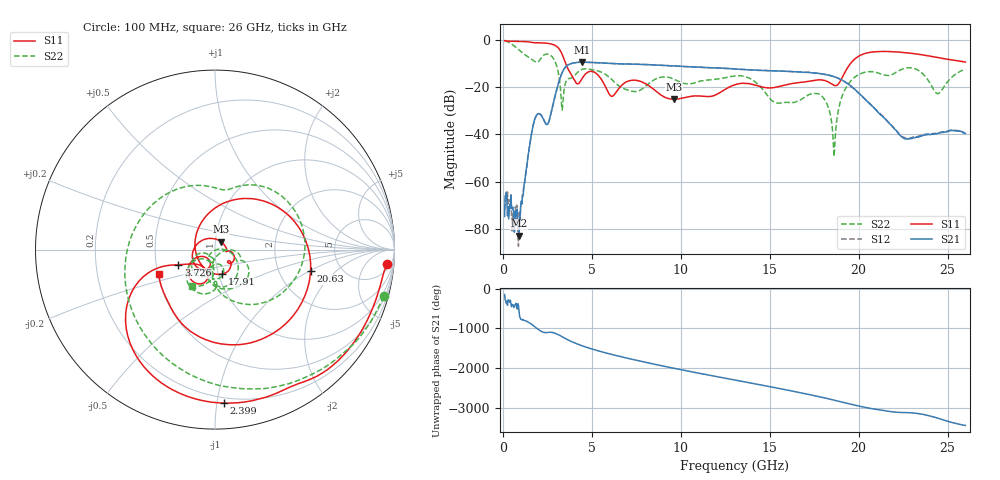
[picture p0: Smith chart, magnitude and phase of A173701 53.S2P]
!  2-Port S-parameters saved by WinCal
! VAR MeasName=S-Parameters (CALIBRATED_DATA) read from VNA (N5245A)
! VAR MeasDate=2017-6-7 10:31:55
! VAR NAME=A173701 53
! VAR FILENAME=A173701 53.S2P
! VAR DATE=2017-6-7 10:31:55
! VAR PHYS_PORTS=1,2
# Hz S DB R 50
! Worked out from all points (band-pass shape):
!   801 points, 100 MHz to 26 GHz, reference 50 ohm
!   highest |S21| = -9.40 dB at 4.438 GHz (marker M1); lowest = -83.0 dB at 909.4 MHz (marker M2)
!   |S21| within 3 dB of the highest: 3.435 GHz to 13.26 GHz (9.823 GHz wide, 118 % of centre)
!   lowest |S11| = -25.1 dB at 9.618 GHz (marker M3), VSWR 1.12, Z = 53.2 + j4.72 ohm
!   |S11| at or under -10 dB: 3.534 GHz to 19.54 GHz (16.01 GHz wide, 139 % of centre)
!   |S22| runs from -49.5 to -0.2 dB; largest |S21 - S12| = 0.0033
!   S11 on the Smith chart (normalised r, x): 100 MHz: 9, -20; 2.399 GHz: 0.16, -1.05; 3.726 GHz: 0.65, -0.12; 17.91 GHz: 1.04, -0.29; 20.63 GHz: 3.02, -1.02; 26 GHz: 0.51, -0.16
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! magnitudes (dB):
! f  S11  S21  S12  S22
! 100 MHz  -0.3  -74.8  -71.8  -0.2
! 909.4 MHz  -0.6  -83.0  -73.2  -4.2
! 1.751 GHz  -1.2  -34.8  -34.7  -8.9
! 2.399 GHz  -1.3  -35.3  -35.2  -6.1
! 2.949 GHz  -2.4  -23.4  -23.3  -9.3
! 3.337 GHz  -6.1  -13.8  -13.8  -29.7
! 3.726 GHz  -13.1  -10.3  -10.3  -16.3
! 4.438 GHz  -16.6  -9.4  -9.4  -12.5
! 7.32 GHz  -17.0  -10.3  -10.2  -21.8
! 8.744 GHz  -22.5  -10.7  -10.7  -16.1
! 9.618 GHz  -25.1  -11.0  -11.0  -16.6
! 13.05 GHz  -18.9  -12.3  -12.3  -15.3
! 15.38 GHz  -20.0  -13.1  -13.1  -26.6
! 17.39 GHz  -17.3  -13.9  -13.9  -22.8
! 17.91 GHz  -16.9  -14.4  -14.3  -23.6
! 18.62 GHz  -19.2  -15.5  -15.6  -49.5
! 19.27 GHz  -13.2  -17.9  -18.0  -20.6
! 20.63 GHz  -5.3  -27.1  -27.0  -13.4
! 21.69 GHz  -4.9  -35.1  -34.9  -15.1
! 23.15 GHz  -5.8  -41.5  -41.2  -12.2
! 24.45 GHz  -7.5  -39.5  -39.4  -22.7
! 26 GHz  -9.3  -39.7  -39.7  -12.4
